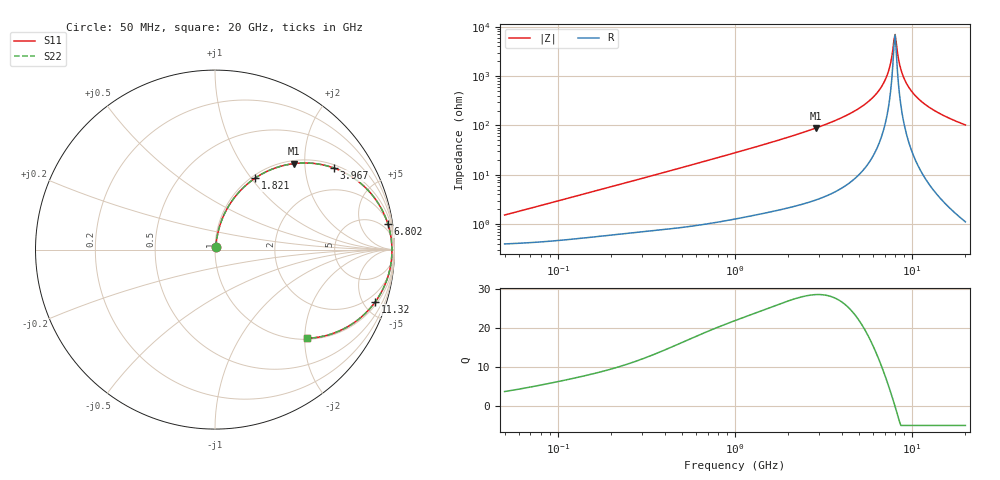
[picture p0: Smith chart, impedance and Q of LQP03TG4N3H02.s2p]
!Murata Part Number: LQP03TG4N3H02
!These Parameters are Measured in Series Mode Connection
!  o--[Z]--o
!Port1  Port2
!  o-------o
!Freq. Start=50[MHz] Stop=20[GHz], 401[Steps]
# Hz S RI R 50
!Freq.(Hz) S11(Real) S11(Imag) S21(Real) S21(Imag) S12(Real) S12(Imag) S22(Real) S22(Imag)
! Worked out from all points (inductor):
!   401 points, 50 MHz to 20 GHz, reference 50 ohm
!   read as one part in series: L = 4.7 nH near 51.52 MHz
!   highest Q = 28.6 at 2.853 GHz (marker M1), where L = 4.92 nH
!   self-resonance near 7.902 GHz
!   S11 on the Smith chart (normalised r, x): 50 MHz: 1.01, +0.03; 1.821 GHz: 1.04, +1.04; 3.967 GHz: 1.11, +2.83; 6.802 GHz: 2, +13; 11.32 GHz: 1.22, -6.06; 20 GHz: 1.02, -2.04
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5e7  0.00418 0.0147  0.9958 -0.0147  0.9958 -0.0147  0.00418 0.0147
1.364002e8  0.0067 0.039  0.9933 -0.039  0.9933 -0.039  0.0067 0.039
3.721004e8  0.0181 0.1018  0.9819 -0.1018  0.9819 -0.1018  0.0181 0.1018
1e9  0.0821 0.2527  0.9179 -0.2527  0.9179 -0.2527  0.0821 0.2527
1.820564e9  0.2224 0.3973  0.7776 -0.3973  0.7776 -0.3973  0.2224 0.3973
2.728004e9  0.4128 0.4751  0.5872 -0.4751  0.5872 -0.4751  0.4128 0.4751
2.853386e9  0.4397 0.4792  0.5603 -0.4792  0.5603 -0.4792  0.4397 0.4792
3.967106e9  0.6612 0.4551  0.3388 -0.4551  0.3388 -0.4551  0.6612 0.4551
5.515528e9  0.8757 0.3045  0.1243 -0.3045  0.1243 -0.3045  0.8757 0.3045
6.217679e9  0.9326 0.2176  0.0674 -0.2176  0.0674 -0.2176  0.9326 0.2176
6.802353e9  0.9629 0.144  0.0371 -0.144  0.0371 -0.144  0.9629 0.144
7.114996e9  0.9735 0.1052  0.0265 -0.1052  0.0265 -0.1052  0.9735 0.1052
7.442007e9  0.981 0.0654  0.019 -0.0654  0.019 -0.0654  0.981 0.0654
7.784049e9  0.9851 0.025  0.0149 -0.025  0.0149 -0.025  0.9851 0.025
8.020766e9  0.986 -0.00208  0.014 0.00208  0.014 0.00208  0.986 -0.00208
8.141811e9  0.9859 -0.0156  0.0141 0.0156  0.0141 0.0156  0.9859 -0.0156
8.644534e9  0.9816 -0.0697  0.0184 0.0697  0.0184 0.0697  0.9816 -0.0697
9.178299e9  0.9714 -0.1228  0.0286 0.1228  0.0286 0.1228  0.9714 -0.1228
1.004137e10  0.9455 -0.1991  0.0545 0.1991  0.0545 0.1991  0.9455 -0.1991
1.131968e10  0.8933 -0.2909  0.1067 0.2909  0.1067 0.2909  0.8933 -0.2909
1.438523e10  0.7451 -0.4261  0.2549 0.4261  0.2549 0.4261  0.7451 -0.4261
2e10  0.5109 -0.4944  0.4891 0.4944  0.4891 0.4944  0.5109 -0.4944
